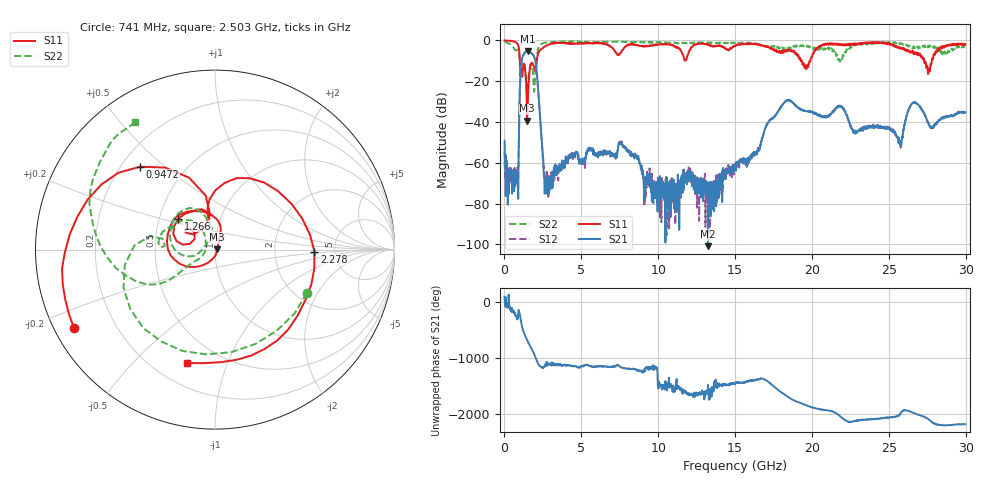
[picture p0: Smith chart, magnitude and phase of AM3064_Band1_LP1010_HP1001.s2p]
# Hz S DB R 50.0
!freq dBS11 angS11 dBS21 angS21 dBS12 angS12 dBS22 angS22
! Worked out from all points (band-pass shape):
!   1600 points, 10 MHz to 29.98 GHz, reference 50 ohm
!   highest |S21| = -5.16 dB at 1.51 GHz (marker M1); lowest = -100.9 dB at 13.24 GHz (marker M2)
!   |S21| within 3 dB of the highest: 1.167 GHz to 1.937 GHz (770.6 MHz wide, 49.7 % of centre)
!   lowest |S11| = -39.4 dB at 1.472 GHz (marker M3), VSWR 1.02, Z = 51.1 + j0.225 ohm
!   |S11| at or under -10 dB: 1.002 GHz to 2.104 GHz (1.103 GHz wide, 71 % of centre); 19.35 GHz to 19.9 GHz (549 MHz wide, 2.8 % of centre); 27.3 GHz to 27.79 GHz (494.1 MHz wide, 1.79 % of centre)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
!   |S22| runs from -25.2 to -0.4 dB; largest |S21 - S12| = 0.0086
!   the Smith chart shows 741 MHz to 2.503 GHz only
!   S11 on the Smith chart (normalised r, x): 741 MHz: 0.06, -0.26; 947.2 MHz: 0.28, +0.42; 1.266 GHz: 0.63, +0.23; 2.278 GHz: 3.48, -0.11; 2.503 GHz: 0.33, -0.73
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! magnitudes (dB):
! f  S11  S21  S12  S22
! 10 MHz  0.0  -49.2  -54.3  -0.4
! 741 MHz  -0.9  -64.9  -66.2  -4.9
! 947.2 MHz  -4.1  -43.5  -43.6  -5.9
! 1.266 GHz  -11.5  -6.7  -6.6  -11.0
! 1.472 GHz  -39.4  -5.2  -5.2  -25.2
! 1.51 GHz  -31.7  -5.2  -5.2  -23.2
! 1.978 GHz  -14.4  -9.1  -9.1  -19.8
! 2.278 GHz  -5.1  -33.4  -33.3  -2.6
! 2.503 GHz  -3.7  -57.7  -57.9  -1.5
! 2.765 GHz  -2.4  -71.5  -66.5  -1.0
! 5.015 GHz  -1.3  -59.1  -59.3  -0.7
! 7.582 GHz  -6.0  -50.8  -49.9  -0.6
! 10 GHz  -2.0  -79.1  -71.7  -1.0
! 13.24 GHz  -2.0  -100.9  -72.3  -1.0
! 15 GHz  -2.7  -61.6  -63.6  -1.4
! 18.3 GHz  -4.9  -29.7  -29.9  -3.6
! 19.99 GHz  -8.4  -35.3  -35.2  -3.3
! 25 GHz  -1.4  -43.2  -43.0  -1.0
! 25.78 GHz  -4.1  -51.8  -51.6  -1.6
! 26.64 GHz  -6.4  -30.6  -30.4  -3.5
! 27.56 GHz  -16.4  -40.3  -40.0  -2.6
! 29.98 GHz  -1.8  -35.3  -35.5  -3.0
